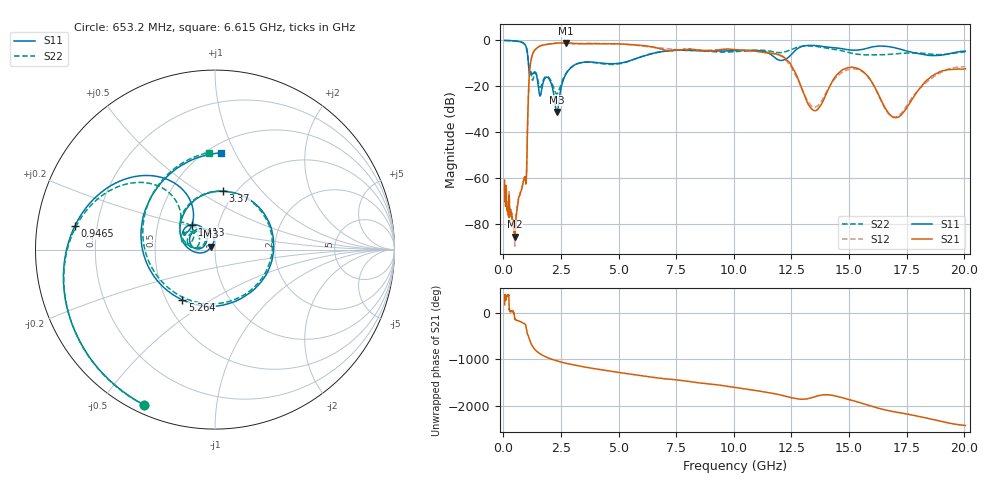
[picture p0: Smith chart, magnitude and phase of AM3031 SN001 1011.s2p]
# Hz S DB R 50
!freq MagS11 AngS11 MagS21 AngS21 MagS12 AngS12 MagS22 AngS22
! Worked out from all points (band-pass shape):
!   1601 points, 50 MHz to 20.05 GHz, reference 50 ohm
!   highest |S21| = -1.06 dB at 2.702 GHz (marker M1); lowest = -85.6 dB at 485.9 MHz (marker M2)
!   |S21| within 3 dB of the highest: 1.372 GHz to 6.93 GHz (5.558 GHz wide, 134 % of centre); 9.4 GHz to 10.12 GHz (715.2 MHz wide, 7.33 % of centre)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
!   lowest |S11| = -31.2 dB at 2.317 GHz (marker M3), VSWR 1.06, Z = 47.8 + j1.58 ohm
!   |S11| at or under -10 dB: 1.082 GHz to 3.238 GHz (2.156 GHz wide, 99.8 % of centre); 4.387 GHz to 4.981 GHz (594.4 MHz wide, 12.7 % of centre)
!   |S22| runs from -23.3 to 0.0 dB; largest |S21 - S12| = 0.068
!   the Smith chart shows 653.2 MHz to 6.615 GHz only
!   S11 on the Smith chart (normalised r, x): 653.2 MHz: 0.04, -0.64; 946.5 MHz: 0.12, +0.08; 1.413 GHz: 0.75, +0.22; 3.37 GHz: 0.88, +0.64; 5.264 GHz: 0.60, -0.38; 6.615 GHz: 0.58, +0.88
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5e7  -0.02 -8.5  -61.01 164.3  -64.43 -11.3  -0.02 -8.3
1.35947e8  -0.05 -22.7  -70.82 -12.7  -71.61 -12.4  -0.03 -22.6
3.696318e8  -0.13 -61.9  -77.28 22.2  -76.15 28.4  -0.13 -62.4
4.858895e8  -0.22 -82.7  -85.60 -130.6  -89.32 162.1  -0.20 -83.0
6.532325e8  -0.44 -114.7  -68.84 -178.7  -68.79 -180.0  -0.43 -114.5
9.465364e8  -2.02 170.6  -59.71 108.5  -59.50 107.7  -2.02 172.2
1.005007e9  -3.48 146.8  -56.94 -20.5  -56.91 -22.0  -3.63 148.9
1.137258e9  -14.88 140.4  -13.26 130.0  -13.31 130.1  -12.13 141.9
1.413263e9  -14.47 132.4  -3.67 -93.2  -3.68 -93.5  -14.34 151.1
1.710794e9  -18.80 176.0  -2.07 163.4  -2.02 162.9  -17.70 174.4
2.317299e9  -31.19 143.2  -1.17 47.8  -1.21 48.0  -23.34 150.2
2.702015e9  -14.86 167.4  -1.06 -2.3  -1.27 -2.4  -14.50 161.8
2.722335e9  -14.51 164.7  -1.08 -4.9  -1.27 -4.9  -14.18 159.8
3.370377e9  -9.67 82.0  -1.46 -70.2  -1.36 -68.1  -9.71 86.5
5.263655e9  -9.52 -122.9  -1.65 141.9  -1.66 142.1  -9.64 -134.4
6.615032e9  -5.36 86.7  -3.17 47.8  -3.07 51.3  -5.32 93.6
7.401857e9  -4.35 9.6  -4.28 7.6  -3.95 3.3  -4.34 26.6
8.76102e9  -4.44 -109.1  -4.43 -76.1  -4.38 -73.1  -4.73 -93.0
1.021551e10  -4.44 119.6  -4.15 -171.6  -4.19 -170.4  -4.81 115.4
1.151657e10  -5.60 -21.6  -5.40 90.2  -5.25 89.5  -4.58 -5.4
1.378533e10  -2.53 -176.4  -28.01 35.4  -26.80 31.5  -2.95 -159.5
2.005e10  -4.65 43.4  -12.41 108.9  -11.44 109.0  -4.96 65.9
